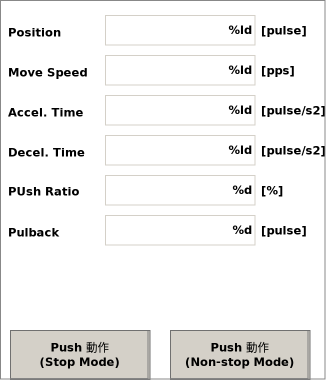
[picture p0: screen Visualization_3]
VISUALIZATION Visualization_3  // 326x380
    Textfield (105,15 150x30), "%ld", text variable: move_prg.target_pos_push
        OnMouseClick: write the text variable via Default, min -2147483648, max 2147483647, format 10000
    Label (5,20 80x25), "Position"
    Label (258,23 50x15), "[pulse]"
    Textfield (105,55 150x30), "%ld", text variable: main.profile_velocity
        OnMouseClick: write the text variable via Default, min 1, max 2500000, format 10000
    Label (5,60 80x25), "Move Speed"
    Label (258,63 50x15), "[pps]"
    Textfield (105,95 150x30), "%ld", text variable: main.profile_acceleration
        OnMouseClick: write the text variable via Default, min 1000, max 1000000000, format 1000000
    Label (5,100 80x25), "Accel. Time"
    Label (258,103 68x15), "[pulse/s2]"
    Textfield (105,135 150x30), "%ld", text variable: main.profile_deceleration
        OnMouseClick: write the text variable via Default, min 1000, max 1000000000, format 1000000
    Label (5,140 80x25), "Decel. Time"
    Label (258,143 66x15), "[pulse/s2]"
    Textfield (105,175 150x30), "%d", text variable: main.push_ratio
        OnMouseClick: write the text variable via Default, min 0, max 100, format 50
    Label (5,179 80x25), "PUsh Ratio"
    Label (258,183 50x15), "[%]"
    Textfield (105,215 150x30), "%d", text variable: main.pull_back
        OnMouseClick: write the text variable via Default, min 0, max 2147483647, format 100
    Label (5,220 80x25), "Pulback"
    Label (258,223 50x15), "[pulse]"
    Button (10,330 140x50), "Push 動作 (Stop Mode)"
        tap move_prg.stop_mode
    Button (170,330 140x50), "Push 動作 (Non-stop Mode)"
        tap move_prg.non_stop_mode
END_VISUALIZATION
